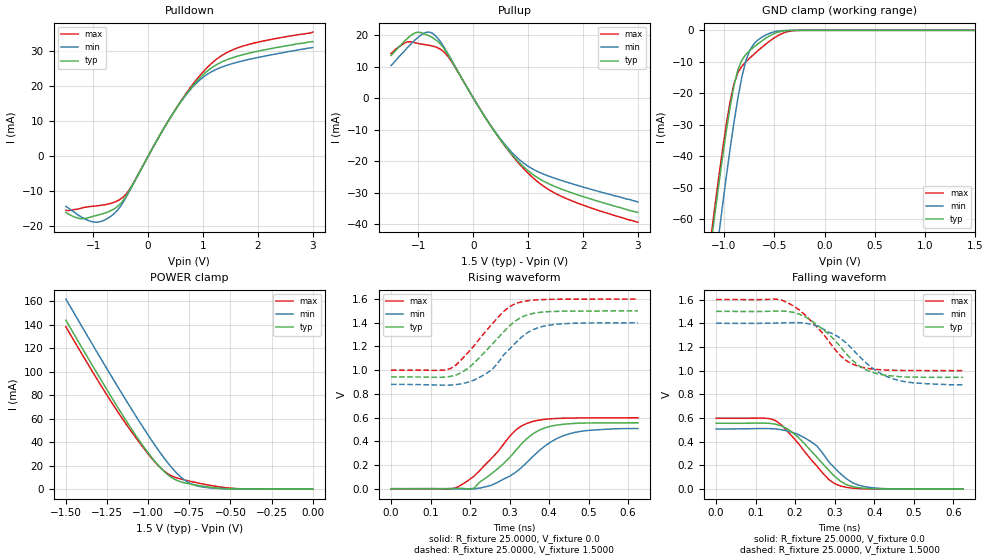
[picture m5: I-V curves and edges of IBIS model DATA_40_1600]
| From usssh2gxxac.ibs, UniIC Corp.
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|   Model DATA_40_1600
[Model]  DATA_40_1600
Model_type I/O
Polarity   Non-Inverting
Enable   Active-High
Vinl =   0.60000000V
Vinh =   0.90000000V
Vmeas =   0.750000000V
Rref =   25.00000000
Vref =   0.75000000V
C_comp   1.6160pF   1.5990pF   1.6430pF
[Temperature Range]   25.0000   95.0000   0.0
[Voltage Range]   1.5000V   1.4000V   1.6000V
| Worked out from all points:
|   slope of the pulldown table from 0 to 0.225 V, typ, clamps not added: 35.8 ohm
|   slope of the pullup table from 0 to 0.225 V, typ, clamps not added: 35.3 ohm
|   GND clamp passes 1 mA (typ) near -0.50 V on its own axis
|   POWER clamp passes 1 mA (typ) near -0.58 V on its own axis
|   rising waveform, R_fixture 25.0000, V_fixture 0.0: 20-80 % time 104ps typ, 113ps min, 96.5ps max; typ from 0 V to 0.556 V
|   rising waveform, R_fixture 25.0000, V_fixture 1.5000: 20-80 % time 96.8ps typ, 90.8ps min, 93.7ps max; typ from 0.943 V to 1.5 V
|   falling waveform, R_fixture 25.0000, V_fixture 0.0: 20-80 % time 94.1ps typ, 87.6ps min, 91.1ps max; typ from 0.556 V to 0 V
|   falling waveform, R_fixture 25.0000, V_fixture 1.5000: 20-80 % time 102ps typ, 109ps min, 95.2ps max; typ from 1.5 V to 0.943 V
[Pulldown]
|Voltage   I(typ)   I(min)   I(max)
-1.5V     -16mA      -14.3mA    -15.4mA
-1.25V    -17.76mA   -17mA      -14.93mA
-1V       -17.11mA   -18.73mA   -14.24mA
-800mV    -16.23mA   -18.22mA   -13.86mA
-600mV    -14.78mA   -16.05mA   -13mA
-350mV    -9.992mA   -10.19mA   -9.704mA
200mV     5.609mA    5.658mA    5.604mA
550mV     14.47mA    14.45mA    14.59mA
850mV     20.7mA     20.32mA    21.19mA
1.15V     25.08mA    23.98mA    26.33mA
1.75V     28.97mA    27.21mA    31.42mA
3V        32.6mA     30.9mA     35.3mA
[Pullup]
|Voltage   I(typ)   I(min)   I(max)
-1.5V     13.5mA     10.3mA     14.1mA
-1.25V    18.14mA    15mA       17.49mA
-1.05V    20.75mA    18.62mA    17.5mA
-900mV    20.45mA    20.57mA    17mA
-750mV    19.21mA    20.61mA    16.54mA
-600mV    17.13mA    17.9mA     15.49mA
-450mV    13.47mA    13.7mA     12.92mA
350mV     -9.677mA   -9.536mA   -9.657mA
900mV     -21.53mA   -20.42mA   -22.09mA
1.25V     -26.1mA    -23.92mA   -27.61mA
1.6V      -28.86mA   -26.12mA   -31.16mA
3V        -36.3mA    -33mA      -39.4mA
[GND_clamp]
|Voltage   I(typ)   I(min)   I(max)
-1.5V     -169mA     -189.1mA   -163.8mA
-1.14V    -70.71mA   -88.3mA    -68.32mA
-1.1V     -60.74mA   -77.66mA   -58.33mA
-1.06V    -51.03mA   -67.22mA   -48.61mA
-1.02V    -41.65mA   -57.06mA   -39.27mA
-940mV    -24.55mA   -37.9mA    -22.88mA
-860mV    -12.39mA   -21.26mA   -13.32mA
-780mV    -7.577mA   -9.433mA   -9.942mA
-740mV    -6.329mA   -6.125mA   -8.71mA
-620mV    -3.273mA   -2.113mA   -5.305mA
-300mV    -11.81uA   -4.878uA   -91.71uA
1.5V      4.577nA    23.6nA     33.33nA
[POWER_clamp]
|Voltage   I(typ)   I(min)   I(max)
-1.5V     143.7mA    161.7mA    138.1mA
-1.22V    77.56mA    95.29mA    73.32mA
-1.12V    55.19mA    72.34mA    52.54mA
-1.02V    34.59mA    50.23mA    33.56mA
-960mV    23.77mA    37.63mA    23.28mA
-900mV    14.66mA    25.9mA     15mA
-840mV    8.415mA    15.63mA    10.28mA
-780mV    5.408mA    7.848mA    7.861mA
-700mV    3.206mA    2.693mA    5.332mA
-600mV    1.29mA     794.5uA    2.681mA
-420mV    69.47uA    44.47uA    238.7uA
0V        4.577nA    6.249nA    39.08nA
[Ramp]
| variable   typ   min   max
dV/dt_r  0.3336/0.1041n   0.3046/0.1129n   0.3589/96.4996p
dV/dt_f  0.3342/0.1019n   0.3119/0.1089n   0.3600/95.1948p
R_load = 25.0000
[Rising Waveform]
R_fixture= 25.0000
V_fixture= 0.0
V_fixture_min= 0.0
V_fixture_max= 0.0
|time   V(typ)   V(min)   V(max)
0s        0V         0V         0V
150ps     2.312mV    -445.7uV   -3.304mV
210ps     3.18mV     -1.232mV   105.6mV
255ps     128.5mV    30.22mV    258.1mV
315ps     319.9mV    136.9mV    493.1mV
360ps     465.2mV    274.7mV    568.7mV
405ps     527.9mV    395.6mV    590mV
450ps     547.6mV    462.1mV    595.9mV
495ps     554.3mV    490.5mV    597.4mV
625ps     556mV      507.7mV    598.1mV
[Rising Waveform]
R_fixture= 25.0000
V_fixture= 1.5000
V_fixture_min= 1.4000
V_fixture_max= 1.6000
|time   V(typ)   V(min)   V(max)
0s        943.1mV    880.2mV    1V
150ps     946.9mV    874.4mV    1.012V
165ps     959.4mV    878.4mV    1.045V
195ps     1.016V     898.2mV    1.149V
255ps     1.215V     1.003V     1.386V
300ps     1.374V     1.178V     1.536V
330ps     1.447V     1.278V     1.577V
360ps     1.479V     1.343V     1.591V
405ps     1.495V     1.382V     1.598V
625ps     1.5V       1.4V       1.6V
[Falling Waveform]
R_fixture= 25.0000
V_fixture= 0.0
V_fixture_min= 0.0
V_fixture_max= 0.0
|time   V(typ)   V(min)   V(max)
0s        556mV      507.6mV    598.1mV
150ps     548.3mV    508.2mV    579.3mV
195ps     473.9mV    476.9mV    436.1mV
240ps     323.6mV    400.5mV    251mV
255ps     269.6mV    364.7mV    194.2mV
285ps     159.1mV    230.3mV    81.51mV
315ps     66mV       129.8mV    26.07mV
345ps     22.07mV    54.89mV    8.88mV
390ps     4.435mV    13.7mV     1.706mV
625ps     0V         0V         0V
[Falling Waveform]
R_fixture= 25.0000
V_fixture= 1.5000
V_fixture_min= 1.4000
V_fixture_max= 1.6000
|time   V(typ)   V(min)   V(max)
0s        1.5V       1.4V       1.6V
150ps     1.503V     1.401V     1.604V
180ps     1.5V       1.404V     1.575V
225ps     1.455V     1.401V     1.47V
255ps     1.388V     1.377V     1.368V
315ps     1.2V       1.273V     1.125V
360ps     1.045V     1.128V     1.036V
405ps     976.2mV    998.9mV    1.01V
450ps     953.6mV    928.4mV    1.003V
625ps     943.1mV    880.4mV    1V
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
